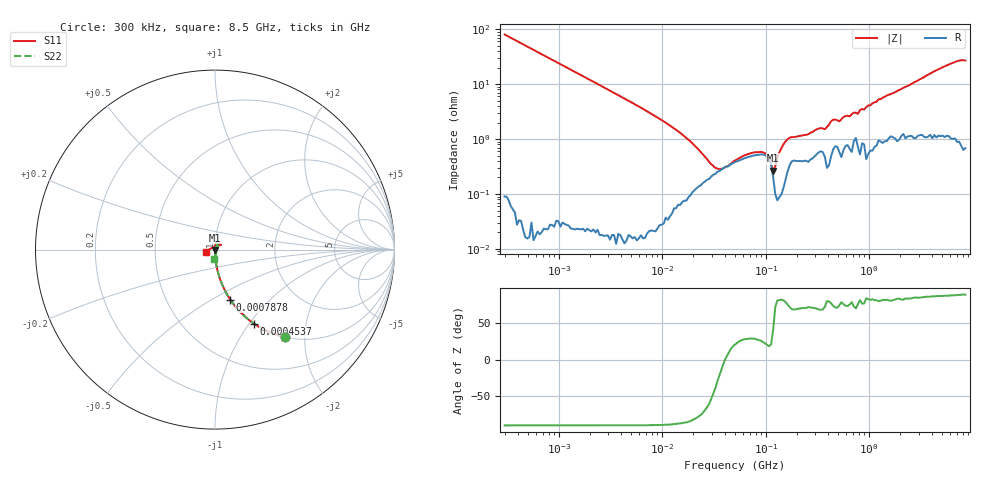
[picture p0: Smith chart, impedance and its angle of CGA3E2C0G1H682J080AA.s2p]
! S-parameter Generated by TDK Corporation
! Copyright(C) 2015 TDK Corporation.
! All Rights Reserved.
! TDK P/N: CGA3E2C0G1H682J080AA (Multilayer Ceramic Chip Capacitors)
! Property: C=6.8nF
! Size(LxWxT): 1.6x0.8x0.8mm, 0.063x0.031x0.031inches
! Model Type: s2p (Touchstone File Format Version 1.0)
! Frequency: DC=Yes Start=0.3MHz Stop=8500MHz 225points Log-sweep
! Note:
! Model Generated on Jun. 23, 2015
! Hash(MD5):
! Port Assignments:
!  1 ---| |--- 2
! Applicable Conditions:
!  Temperature = 25 degC
!  DC Bias Voltage = 0 V
!  Small Signal Operation
! Terms and conditions regarding TDK Simulation Models
! (1)This simulation model is being provided solely for informational purposes. Please refer to the specifications of the products in terms of detailed characteristics of such products.
! (2)In no event shall TDK Corporation of any of its subsidiaries be liable for any loss or damage arising, directly or indirectly,
!  From any information contained in this simulation model, including, but not limited to loss or damages arising from any inaccuracies, omissions or errors in connection with such information.
! (3)Any and all copyrights on this simulation model are owned by TDK Corporation.
!  Duplication or redistribution of this simulation model without prior written permission from TDK Corporation is prohibited.
! (4)This simulation model is subject to any modification or change without any prior notice.
! (5)Neither TDK Corporation nor any of its subsidiaries shall make any warranty, express or implied,
!  Including but not limited to the correctness, implied warranties of merchantability and fitness for a particular purpose with respect to this simulation models.
! (6)The use of this simulation model shall be deemed to have consented to the terms and conditions hereof.
# MHz S MA R 50
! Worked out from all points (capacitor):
!   224 points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, 300 kHz to 8.5 GHz, reference 50 ohm
!   read as one part in series: C = 6.62 nF near 314.1 kHz
!   lowest |Z| = 267 mohm at 118.2 MHz (marker M1)
!   series resonance near 40.61 MHz, so ESL is about 2.3 nH
!   S11 on the Smith chart (normalised r, x): 300 kHz: 1.00, -1.61; 453.7 kHz: 1.00, -1.06; 787.8 kHz: 1.00, -0.61; 8.5 GHz: 0.91, -0.02
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0.3  0.6257 -51.2  0.78 38.7  0.78 38.8  0.6257 -51.3
0.4537435  0.468 -62.1  0.8832 27.9  0.8834 28.0  0.4676 -62.1
0.7877636  0.2912 -73.0  0.9563 17.0  0.9565 17.0  0.291 -73.0
1.72111  0.1378 -82.0  0.9903 7.9  0.9902 8.0  0.1378 -82.0
9.430415  0.02381 -88.5  0.9994 1.3  0.9995 1.3  0.02375 -87.6
31.16253  0.003177 -87.3  0.9973 0.0  0.9976 0.1  0.00572 -49.6
45.01492  0.0001247 -133.9  0.9956 -0.2  0.9963 -0.1  0.006119 -29.4
51.67171  0.0007408 107.5  0.9948 -0.3  0.9954 -0.2  0.006613 -27.7
102.9757  0.0004025 -11.8  0.9917 -0.4  0.9927 -0.4  0.007908 -66.7
118.2037  0.001986 -109.3  0.9946 -0.4  0.9951 -0.4  0.006059 -106.5
283.1228  0.003615 -137.8  0.9885 -1.5  0.9892 -1.4  0.003388 126.1
491.5417  0.0006556 122.3  0.9855 -2.4  0.9865 -2.3  0.001536 42.3
538.8791  0.00357 -118.4  0.9877 -2.5  0.9889 -2.5  0.00689 114.4
618.5683  0.0009502 -122.3  0.9847 -2.8  0.9859 -2.8  0.004784 64.3
743.4462  0.005011 -31.0  0.9844 -3.2  0.9854 -3.2  0.008055 29.4
778.4218  0.003405 -20.1  0.9878 -3.2  0.9884 -3.2  0.001864 41.4
815.0429  0.0008537 82.6  0.9901 -3.6  0.9903 -3.6  0.007592 76.3
893.5346  0.005066 15.5  0.9871 -3.9  0.9869 -3.8  0.002407 -61.0
1025.67  0.001202 -17.1  0.9856 -4.6  0.9873 -4.6  0.003711 158.0
1551.304  0.008557 39.5  0.9823 -6.9  0.9832 -6.7  0.009671 73.2
7753.325  0.01641 105.6  0.98 -32.5  0.9799 -32.2  0.01235 -2.9
8500  0.051 -166.6  0.9792 -35.4  0.979 -35.5  0.05296 -93.8
